(* Logix 5000 AddOnInstructionDefinition export AMCI_SMD34E2_Jog_CCW; software revision 20.03 *)

ADD_ON_INSTRUCTION AMCI_SMD34E2_Jog_CCW   (* revision 1.0, vendor AMCI *)
VAR_INPUT
   Programmed_Speed : DINT; {required}
   Acceleration : INT; {required}
   Deceleration : INT; {required}
   Jerk : INT;
END_VAR
VAR_OUTPUT
   Jog_CCW_Occurring : BOOL; {access Read Only, visible}
END_VAR
VAR_IN_OUT
   AMCI_SMD34E2_output_data : _000A:SMD34E2_788832CB:O:0; {required}
END_VAR
VAR
   Upper_Result_X_1000 : DINT;
   command_data_block : INT[10];
        [0]   // Command Bits MSW
        [1]   // Command Bits LSW
        [2]   // Upper Target Position
        [3]   // Lower Target Position
        [4]   // Upper Programmed Speed
        [5]   // Lower Programmed Speed
END_VAR

ROUTINE Logic   (* ladder *)
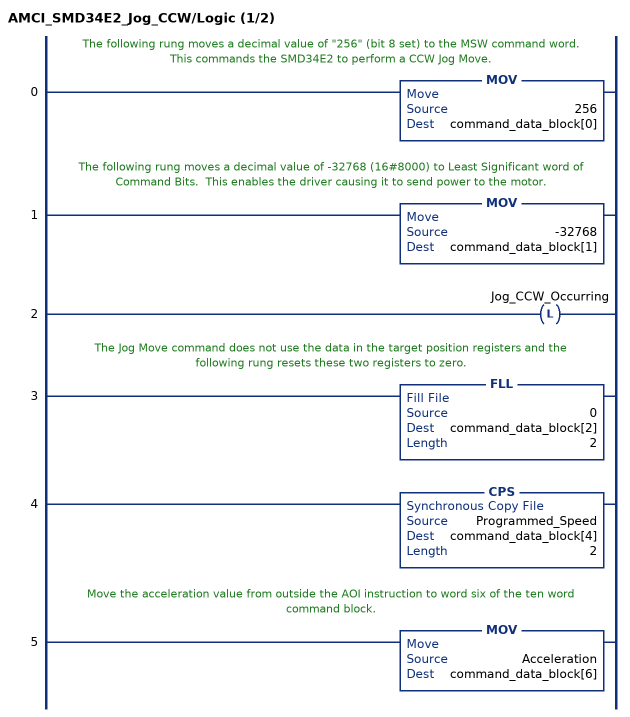
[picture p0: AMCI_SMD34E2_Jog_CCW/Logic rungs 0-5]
   // The following rung moves a decimal value of "256" (bit 8 set) to the MSW command word.  This commands the SMD34E2 to perform a CCW Jog Move.
   0: MOV(256,command_data_block[0]);
   // The following rung moves a decimal value of -32768 (16#8000) to Least Significant word of Command Bits.  This enables the driver causing it to send power to the motor.
   1: MOV(-32768,command_data_block[1]);
   2: OTL(Jog_CCW_Occurring);
   // The Jog Move command does not use the data in the target position registers and the following rung resets these two registers to zero.
   3: FLL(0,command_data_block[2],2);
   4: CPS(Programmed_Speed,command_data_block[4],2);
   // Move the acceleration value from outside the AOI instruction to word six of the ten word command block.
   5: MOV(Acceleration,command_data_block[6]);
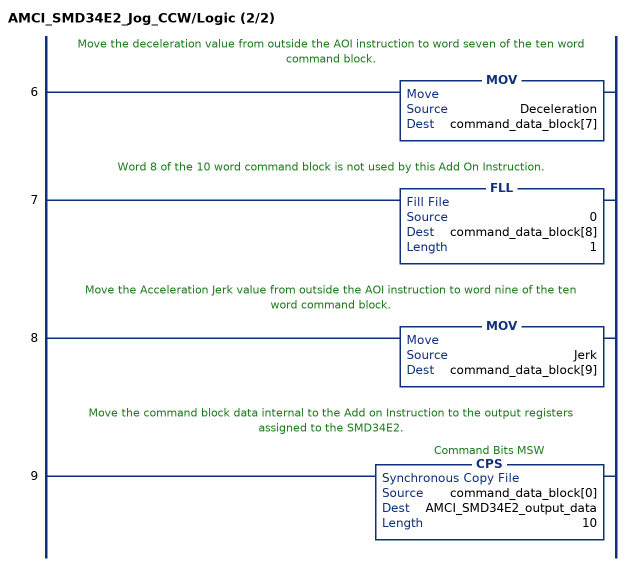
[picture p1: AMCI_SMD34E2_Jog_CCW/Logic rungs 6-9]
   // Move the deceleration value from outside the AOI instruction to word seven of the ten word command block.
   6: MOV(Deceleration,command_data_block[7]);
   // Word 8 of the 10 word command block is not used by this Add On Instruction.
   7: FLL(0,command_data_block[8],1);
   // Move the Acceleration Jerk value from outside the AOI instruction to word nine of the ten word command block.
   8: MOV(Jerk,command_data_block[9]);
   // Move the command block data internal to the Add on Instruction to the output registers assigned to the SMD34E2.
   9: CPS(command_data_block[0],AMCI_SMD34E2_output_data,10);
END_ROUTINE
END_ADD_ON_INSTRUCTION
